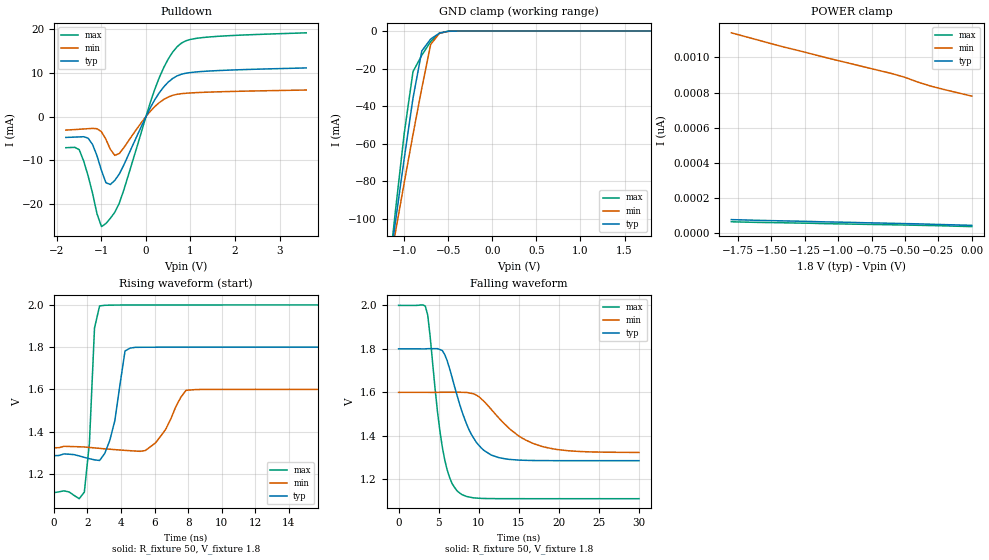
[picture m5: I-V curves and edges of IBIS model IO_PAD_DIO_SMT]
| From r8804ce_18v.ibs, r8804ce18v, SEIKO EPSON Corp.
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[Model]   IO_PAD_DIO_SMT
Model_type I/O_open_drain
Enable Active-High
Polarity Non-Inverting
Vinh=1.6
Vinl=0.32
Vref=2.0
Vmeas=0.90
Rref=5000
C_comp   2.5p   2.0p   3.0p
[Temperature Range] 25   105   -40
[Voltage Range]   1.8   1.6   2.0
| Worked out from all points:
|   slope of the pulldown table from 0 to 0.27 V, typ, clamps not added: 54.4 ohm
|   GND clamp passes 1 mA (typ) near -0.59 V on its own axis
|   falling waveform, R_fixture 50, V_fixture 1.8: 20-80 % time 2.92ns typ, 4.96ns min, 1.74ns max; typ from 1.8 V to 1.29 V
|   rising waveform, R_fixture 50, V_fixture 1.8: 20-80 % time 650ps typ, 1.08ns min, 339ps max; typ from 1.29 V to 1.8 V
[Pulldown]
-1.8V     -4.763mA   -3.077mA   -7.1mA
-1.5V     -4.644mA   -2.906mA   -7.544mA
-1.2V     -6.372mA   -2.699mA   -17.48mA
-1V       -12.3mA    -3.456mA   -25.07mA
-900mV    -15.07mA   -5.196mA   -24.38mA
-800mV    -15.48mA   -7.459mA   -23.19mA
-600mV    -13.11mA   -8.434mA   -19.76mA
200mV     3.863mA    2.284mA    6.265mA
500mV     7.84mA     4.449mA    13.11mA
700mV     9.268mA    5.071mA    15.9mA
1.3V      10.29mA    5.52mA     18.02mA
3.6V      11.07mA    6.04mA     19.07mA
[GND Clamp]
-1.8V     -342.6mA   -297.5mA   -403.5mA
-1.2V     -136mA     -134.3mA   -139.6mA
-1.1V     -101.9mA   -107.4mA   -96.16mA
-1V       -68.05mA   -80.95mA   -54.68mA
-900mV    -35.72mA   -55.09mA   -21.63mA
-800mV    -10.59mA   -30.37mA   -12.89mA
-700mV    -4.3mA     -7.208mA   -5.615mA
-600mV    -1.094mA   -1.181mA   -1.208mA
-500mV    -109.6uA   -173.5uA   -67.33uA
-400mV    -6.015uA   -18.81uA   -1.378uA
1.8V      42.97pA    815.6pA    32.23pA
[POWER Clamp]
-1.8V     75.6pA     1.14nA     63.32pA
-1.4V     68.1pA     1.058nA    57.41pA
-1.1V     62.64pA    1.001nA    52.52pA
-600mV    54.57pA    908.3pA    46.1pA
-500mV    52.81pA    886.5pA    44.74pA
-400mV    51.44pA    858.4pA    43.14pA
-300mV    49.06pA    835.1pA    41.67pA
0V        42.97pA    779.6pA    35.81pA
[Falling Waveform]
R_fixture=50
V_fixture=1.8
V_fixture_min=1.6
V_fixture_max=2.0
0s        1.8V       1.6V       2V
3.333ns   1.8V       1.6V       1.997V
3.636ns   1.801V     1.6V       1.955V
5.455ns   1.793V     1.6V       1.349V
6.364ns   1.709V     1.6V       1.209V
7.576ns   1.551V     1.6V       1.139V
9.697ns   1.37V      1.588V     1.114V
12.42ns   1.301V     1.486V     1.111V
18.18ns   1.286V     1.348V     1.111V
30ns      1.286V     1.324V     1.111V
[Rising Waveform]
R_fixture=50
V_fixture=1.8
V_fixture_min=1.6
V_fixture_max=2.0
0s        1.286V     1.324V     1.111V
1.818ns   1.278V     1.327V     1.114V
2.121ns   1.272V     1.325V     1.345V
2.424ns   1.266V     1.323V     1.89V
2.727ns   1.263V     1.321V     1.995V
3.333ns   1.358V     1.317V     1.999V
4.545ns   1.795V     1.31V      2V
6.061ns   1.8V       1.347V     2V
7.879ns   1.8V       1.596V     2V
30ns      1.8V       1.6V       2V
[Ramp]
R_load=50
dV/dt_r   3.085E-1/6.093E-10   1.659E-1/1.075E-9   5.334E-1/2.975E-10
dV/dt_f   3.085E-1/2.922E-9   1.657E-1/4.952E-9   5.334E-1/1.735E-9
|[End   IO_PAD_DIO_SMT
